FUNCTION_BLOCK Example31_extendedfeedback // any flyway configuration 50 xbots - PMC_ConfigFBStreamExtended, PMC_ReadStreamFeedbackExtended, PMC_ReadXbotSpeed
VAR_INPUT
	Execute : BOOL;
END_VAR
VAR_OUTPUT
END_VAR
VAR_IN_OUT
	PM_Controller : PMControllerType;	// the planar motor controller to use
END_VAR
VAR
	XbotIDs : ARRAY[0..149] OF USINT;
	PMC_ConfigFBStreamExtended1 : PMC_ConfigFBStreamExtended;
	PMC_ReadXbot31X : PMC_ReadStreamFeedbackExtended;
	PMC_ReadXbot31Y : PMC_ReadStreamFeedbackExtended;
	PMC_ReadXbot31Z : PMC_ReadStreamFeedbackExtended;
	PMC_ReadXbot31Speed : PMC_ReadXbotSpeed;
	PMC_ReadXbot42X : PMC_ReadStreamFeedbackExtended;
	PMC_ReadXbot42Y : PMC_ReadStreamFeedbackExtended;
	PMC_ReadXbot42Z : PMC_ReadStreamFeedbackExtended;
	PMC_ReadXbot42Speed : PMC_ReadXbotSpeed;
	PMC_ReadXbot50X : PMC_ReadStreamFeedbackExtended;
	PMC_ReadXbot50Y : PMC_ReadStreamFeedbackExtended;
	PMC_ReadXbot50Z : PMC_ReadStreamFeedbackExtended;
	PMC_ReadXbot50Speed : PMC_ReadXbotSpeed;
	PMC_ReadXbotAnyX : PMC_ReadStreamFeedbackExtended;
	PMC_ReadXbotAnyY : PMC_ReadStreamFeedbackExtended;
	PMC_ReadXbotAnyZ : PMC_ReadStreamFeedbackExtended;
	PMC_ReadXbotAnySpeed : PMC_ReadXbotSpeed;
	X31 : REAL;
	Y31 : REAL;
	Z31 : REAL;
	X42 : REAL;
	Y42 : REAL;
	Z42 : REAL;
	X50 : REAL;
	Y50 : REAL;
	Z50 : REAL;
	AnyXID : USINT := 1;
	XAny : REAL;
	YAny : REAL;
	ZAny : REAL;
END_VAR

// any flyway configuration 50 xbots - PMC_ConfigFBStreamExtended, PMC_ReadStreamFeedbackExtended, PMC_ReadXbotSpeed

//setup extended feedback streaming
XbotIDs[0] := 1;XbotIDs[1] := 2;XbotIDs[2] := 3;XbotIDs[3] := 4;XbotIDs[4] := 5;XbotIDs[5] := 6;XbotIDs[6] := 7;XbotIDs[7] := 8;XbotIDs[8] := 9;XbotIDs[9] := 10;
XbotIDs[10] := 11;XbotIDs[11] := 12;XbotIDs[12] := 13;XbotIDs[13] := 14;XbotIDs[14] := 15;XbotIDs[15] := 16;XbotIDs[16] := 17;XbotIDs[17] := 18;XbotIDs[18] := 19;XbotIDs[19] := 20;
XbotIDs[20] := 21;XbotIDs[21] := 22;XbotIDs[22] := 23;XbotIDs[23] := 24;XbotIDs[24] := 25;XbotIDs[25] := 26;XbotIDs[26] := 27;XbotIDs[27] := 28;XbotIDs[28] := 29;XbotIDs[29] := 30;
XbotIDs[30] := 31;XbotIDs[31] := 32;XbotIDs[32] := 33;XbotIDs[33] := 34;XbotIDs[34] := 35;XbotIDs[35] := 36;XbotIDs[36] := 37;XbotIDs[37] := 38;XbotIDs[38] := 39;XbotIDs[39] := 40;
XbotIDs[40] := 41;XbotIDs[41] := 42;XbotIDs[42] := 43;XbotIDs[43] := 44;XbotIDs[44] := 45;XbotIDs[45] := 46;XbotIDs[46] := 47;XbotIDs[47] := 48;XbotIDs[48] := 49;XbotIDs[49] := 50;
PMC_ConfigFBStreamExtended1(Execute := Execute,nXbots := 50,XbotID := XbotIDs,PM_Controller := PM_Controller);

//read position/speed of xbot 31
PMC_ReadXbot31X(Enable := PMC_ConfigFBStreamExtended1.Done,XbotID := 31,XBotAxisID := 1,FeedbackValue => X31,PM_Controller := PM_Controller);
PMC_ReadXbot31Y(Enable := PMC_ConfigFBStreamExtended1.Done,XbotID := 31,XBotAxisID := 2,FeedbackValue => Y31,PM_Controller := PM_Controller);
PMC_ReadXbot31Z(Enable := PMC_ConfigFBStreamExtended1.Done,XbotID := 31,XBotAxisID := 3,FeedbackValue => Z31,PM_Controller := PM_Controller);
PMC_ReadXbot31Speed(Enable := PMC_ConfigFBStreamExtended1.Done,FeedbackType := 1,ID := 31,PM_Controller := PM_Controller);

//read position/speed of xbot 42
PMC_ReadXbot42X(Enable := PMC_ConfigFBStreamExtended1.Done,XbotID := 42,XBotAxisID := 1,FeedbackValue => X42,PM_Controller := PM_Controller);
PMC_ReadXbot42Y(Enable := PMC_ConfigFBStreamExtended1.Done,XbotID := 42,XBotAxisID := 2,FeedbackValue => Y42,PM_Controller := PM_Controller);
PMC_ReadXbot42Z(Enable := PMC_ConfigFBStreamExtended1.Done,XbotID := 42,XBotAxisID := 3,FeedbackValue => Z42,PM_Controller := PM_Controller);
PMC_ReadXbot42Speed(Enable := PMC_ConfigFBStreamExtended1.Done,FeedbackType := 1,ID := 42,PM_Controller := PM_Controller);

//read position/speed of xbot 50
PMC_ReadXbot50X(Enable := PMC_ConfigFBStreamExtended1.Done,XbotID := 50,XBotAxisID := 1,FeedbackValue => X50,PM_Controller := PM_Controller);
PMC_ReadXbot50Y(Enable := PMC_ConfigFBStreamExtended1.Done,XbotID := 50,XBotAxisID := 2,FeedbackValue => Y50,PM_Controller := PM_Controller);
PMC_ReadXbot50Z(Enable := PMC_ConfigFBStreamExtended1.Done,XbotID := 50,XBotAxisID := 3,FeedbackValue => Z50,PM_Controller := PM_Controller);
PMC_ReadXbot50Speed(Enable := PMC_ConfigFBStreamExtended1.Done,FeedbackType := 1,ID := 50,PM_Controller := PM_Controller);

//read position/speed of any xbot
PMC_ReadXbotAnyX(Enable := PMC_ConfigFBStreamExtended1.Done,XbotID := AnyXID,XBotAxisID := 1,FeedbackValue => XAny,PM_Controller := PM_Controller);
PMC_ReadXbotAnyY(Enable := PMC_ConfigFBStreamExtended1.Done,XbotID := AnyXID,XBotAxisID := 2,FeedbackValue => YAny,PM_Controller := PM_Controller);
PMC_ReadXbotAnyZ(Enable := PMC_ConfigFBStreamExtended1.Done,XbotID := AnyXID,XBotAxisID := 3,FeedbackValue => ZAny,PM_Controller := PM_Controller);
PMC_ReadXbotAnySpeed(Enable := PMC_ConfigFBStreamExtended1.Done,FeedbackType := 1,ID := AnyXID,PM_Controller := PM_Controller);

END_FUNCTION_BLOCK
